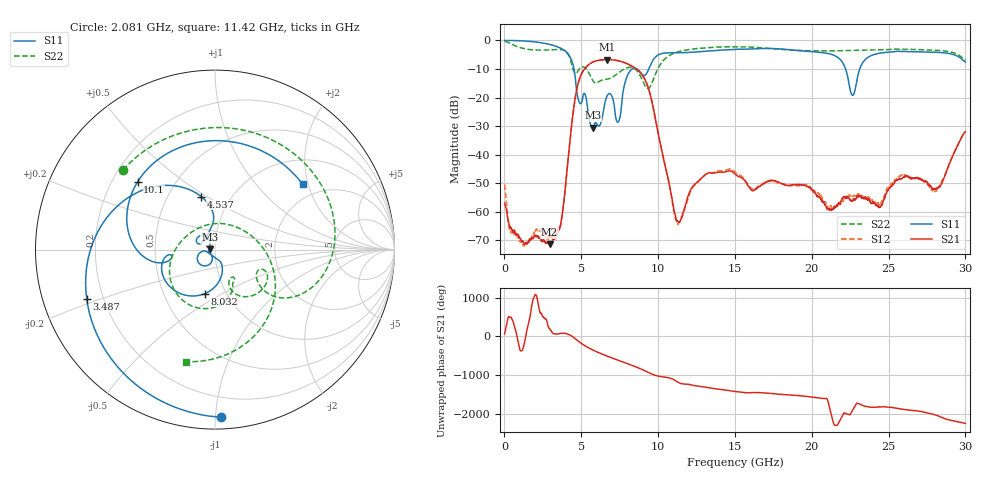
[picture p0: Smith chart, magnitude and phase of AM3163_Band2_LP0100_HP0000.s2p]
!Agilent Technologies,E8364B,MY43040894,A.07.50.67
!Agilent E8364B: A.07.50.67
!Date: Thursday, August 20, 2020 12:05:30
!Correction: S11(Full 2 Port(1,2))
!S21(Full 2 Port(1,2))
!S12(Full 2 Port(1,2))
!S22(Full 2 Port(1,2))
!S2P File: Measurements: S11, S21, S12, S22:
# Hz S  dB  R 50
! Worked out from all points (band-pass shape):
!   3201 points, 10 MHz to 30 GHz, reference 50 ohm
!   highest |S21| = -6.70 dB at 6.692 GHz (marker M1); lowest = -71.4 dB at 2.934 GHz (marker M2)
!   |S21| within 3 dB of the highest: 5.255 GHz to 8.5 GHz (3.245 GHz wide, 47.2 % of centre)
!   lowest |S11| = -30.5 dB at 5.746 GHz (marker M3), VSWR 1.06, Z = 47.1 + j0.192 ohm
!   |S11| at or under -10 dB: 4.525 GHz to 8.31 GHz (3.785 GHz wide, 59 % of centre); 8.64 GHz to 9.392 GHz (752.3 MHz wide, 8.34 % of centre); 22.2 GHz to 23.12 GHz (919.2 MHz wide, 4.06 % of centre)
!   |S22| runs from -16.8 to -0.3 dB; largest |S21 - S12| = 0.0036
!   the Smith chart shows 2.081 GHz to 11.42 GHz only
!   S11 on the Smith chart (normalised r, x): 2.081 GHz: 0.07, -1.03; 3.487 GHz: 0.14, -0.18; 4.537 GHz: 0.73, +0.47; 8.032 GHz: 0.79, -0.42; 10.1 GHz: 0.31, +0.35; 11.42 GHz: 1.59, +1.85
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1e7  -0.02 -3.0  -56.94 65.2  -50.43 1.7  -0.26 -10.9
6.754031e8  -0.06 -27.8  -66.80 -148.8  -67.61 -48.7  -1.85 -95.6
2.081184e9  -0.59 -88.0  -68.76 -24.0  -66.02 -34.1  -3.38 139.1
2.934025e9  -1.39 -128.3  -71.38 -154.6  -68.90 30.7  -3.31 80.0
3.486966e9  -2.32 -158.9  -66.98 67.5  -66.17 71.0  -3.18 40.2
4.536616e9  -10.31 104.5  -22.58 -35.7  -22.57 -36.1  -11.03 -34.4
5.014581e9  -21.85 152.6  -11.70 178.1  -11.71 177.8  -9.31 -34.0
5.745588e9  -30.51 176.1  -7.59 12.3  -7.61 12.2  -14.06 -67.1
6.692147e9  -19.31 -123.0  -6.70 -147.2  -6.70 -147.4  -13.55 -61.9
7.404409e9  -28.57 -119.3  -7.10 107.2  -7.13 107.1  -11.43 -71.8
8.032325e9  -11.97 -103.1  -8.27 15.7  -8.28 15.8  -9.50 -100.8
1.000979e10  -5.08 147.0  -32.70 58.6  -32.60 57.3  -9.65 -15.3
1.010351e10  -4.83 138.7  -35.18 51.9  -35.12 50.4  -8.74 -24.4
1.142494e10  -4.30 36.8  -63.38 -125.1  -62.97 -128.6  -3.81 -104.6
1.32712e10  -3.71 -69.7  -46.39 118.1  -46.33 123.1  -2.51 -170.9
1.5005e10  -3.13 -143.4  -46.75 20.6  -46.01 21.7  -2.21 130.9
1.77041e10  -2.91 94.1  -49.38 -43.1  -49.59 -45.2  -2.99 30.1
2.000958e10  -3.94 -28.3  -52.26 -121.9  -52.41 -121.9  -3.64 -51.0
2.266182e10  -19.22 -108.0  -56.18 -98.9  -54.42 118.7  -3.51 -125.9
2.500479e10  -4.12 -151.4  -52.25 -20.9  -51.31 -24.4  -3.21 176.7
2.812562e10  -4.17 110.0  -51.84 127.2  -52.60 127.8  -3.46 93.3
3e10  -7.53 38.5  -31.96 -78.7  -31.96 -78.8  -7.00 35.5
